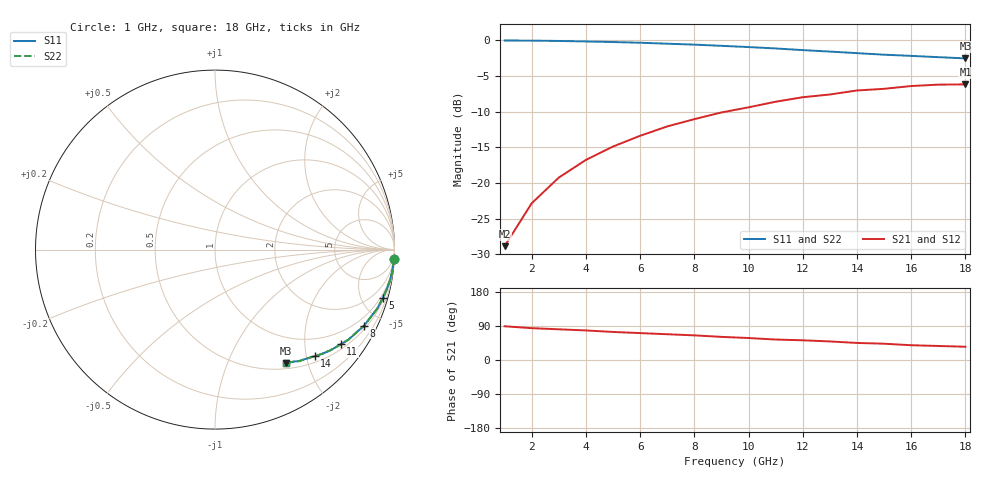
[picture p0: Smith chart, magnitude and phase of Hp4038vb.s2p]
!HPND-4038 beam lead PIN diode
!Series configuration S-parameters Vr= 10 V.  Last updated 10/3/97
# mhz s ma r 50
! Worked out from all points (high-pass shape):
!   18 points, 1 GHz to 18 GHz, reference 50 ohm
!   highest |S21| = -6.18 dB at 18 GHz (marker M1); lowest = -28.9 dB at 1 GHz (marker M2)
!   |S21| within 3 dB of the highest: 10.28 GHz to end of sweep
!   lowest |S11| = -2.5 dB at 18 GHz (marker M3), VSWR 6.91, Z = 28.8 - j82.7 ohm
!   |S11| at or under -10 dB: nowhere
!   |S22| runs from -2.5 to 0.0 dB; largest |S21 - S12| = 0
!   S11 on the Smith chart (normalised r, x): 1 GHz: 1, -38; 5 GHz: 0.70, -7.05; 8 GHz: 0.62, -4.08; 11 GHz: 0.63, -2.87; 14 GHz: 0.61, -2.15; 18 GHz: 0.58, -1.65
1000  0.998 -3.0  0.036 89.0  0.036 89.0  0.998 -3.0
2000  0.995 -7.0  0.072 84.0  0.072 84.0  0.995 -7.0
3000  0.99 -10.0  0.109 81.0  0.109 81.0  0.99 -10.0
4000  0.982 -13.0  0.145 78.0  0.145 78.0  0.982 -13.0
5000  0.973 -16.0  0.18 74.0  0.18 74.0  0.973 -16.0
6000  0.962 -20.0  0.214 71.0  0.214 71.0  0.962 -20.0
7000  0.947 -23.0  0.249 68.0  0.249 68.0  0.947 -23.0
8000  0.933 -27.0  0.28 65.0  0.28 65.0  0.933 -27.0
9000  0.915 -30.0  0.312 61.0  0.312 61.0  0.915 -30.0
10000  0.897 -34.0  0.339 58.0  0.339 58.0  0.897 -34.0
11000  0.877 -37.0  0.371 54.0  0.371 54.0  0.877 -37.0
12000  0.854 -41.0  0.399 52.0  0.399 52.0  0.854 -41.0
13000  0.834 -44.0  0.417 49.0  0.417 49.0  0.834 -44.0
14000  0.813 -47.0  0.445 45.0  0.445 45.0  0.813 -47.0
15000  0.793 -50.0  0.457 43.0  0.457 43.0  0.793 -50.0
16000  0.778 -53.0  0.478 39.0  0.478 39.0  0.778 -53.0
17000  0.762 -55.0  0.489 37.0  0.489 37.0  0.762 -55.0
18000  0.747 -58.0  0.491 35.0  0.491 35.0  0.747 -58.0
